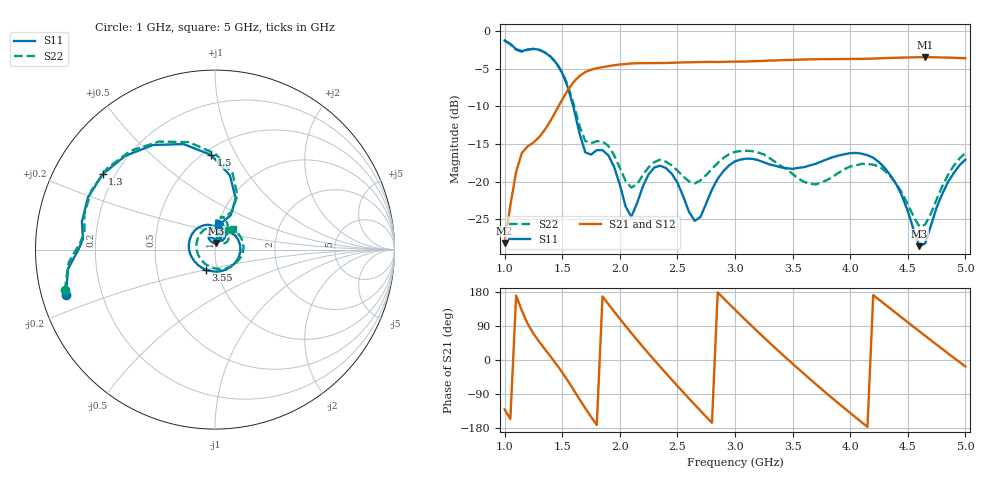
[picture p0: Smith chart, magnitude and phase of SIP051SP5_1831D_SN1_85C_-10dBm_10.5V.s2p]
# GHz  S  dB  R  50
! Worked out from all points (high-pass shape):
!   81 points, 1 GHz to 5 GHz, reference 50 ohm
!   highest |S21| = -3.44 dB at 4.65 GHz (marker M1); lowest = -28.2 dB at 1 GHz (marker M2)
!   |S21| within 3 dB of the highest: 1.618 GHz to end of sweep
!   lowest |S11| = -28.6 dB at 4.6 GHz (marker M3), VSWR 1.08, Z = 50.5 + j3.71 ohm
!   |S11| at or under -10 dB: 1.596 GHz to end of sweep
!   |S22| runs from -26.0 to -1.2 dB; largest |S21 - S12| = 0.002
!   S11 on the Smith chart (normalised r, x): 1 GHz: 0.07, -0.15; 1.3 GHz: 0.15, +0.30; 1.5 GHz: 0.55, +0.80; 3.55 GHz: 0.88, -0.20; 5 GHz: 0.99, +0.28
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1  -1.21 -163.0  -28.17 -130.3  -28.21 -130.4  -1.24 -164.9
1.15  -2.64 175.4  -16.18 129.9  -16.16 130.0  -2.71 172.8
1.3  -2.45 146.1  -14.08 48.2  -14.09 48.2  -2.47 142.9
1.5  -5.55 92.3  -9.08 -32.6  -9.06 -32.7  -5.44 89.8
1.7  -16.09 75.4  -5.42 -127.1  -5.41 -127.2  -14.57 73.1
1.85  -15.81 81.9  -4.76 167.8  -4.75 167.9  -14.67 75.0
2.05  -23.28 68.8  -4.36 89.9  -4.34 89.9  -19.88 63.5
2.2  -20.64 109.1  -4.23 34.8  -4.23 34.9  -19.12 86.2
2.35  -17.88 83.7  -4.22 -17.6  -4.20 -17.6  -17.08 71.2
2.6  -24.00 51.2  -4.12 -101.4  -4.11 -101.4  -19.96 53.7
2.8  -21.06 79.0  -4.07 -165.7  -4.05 -165.8  -18.29 59.2
3  -17.29 36.4  -4.03 132.8  -4.02 132.8  -16.04 32.5
3.25  -17.43 -32.7  -3.93 59.7  -3.92 59.7  -16.38 -14.4
3.4  -18.09 -75.8  -3.83 17.6  -3.83 17.5  -17.93 -48.3
3.55  -18.16 -115.2  -3.77 -23.4  -3.75 -23.5  -19.58 -90.4
3.7  -17.63 -150.1  -3.71 -63.3  -3.71 -63.3  -20.37 -144.7
3.85  -16.74 177.7  -3.69 -102.0  -3.68 -102.1  -19.34 163.4
4.05  -16.18 136.1  -3.67 -152.0  -3.65 -152.1  -17.84 106.6
4.35  -19.18 78.2  -3.54 135.3  -3.54 135.3  -19.31 45.7
4.6  -28.59 80.5  -3.44 75.9  -3.44 75.8  -25.96 47.2
4.65  -28.23 102.9  -3.44 64.0  -3.44 64.0  -25.73 61.8
5  -17.08 83.7  -3.57 -17.0  -3.58 -17.0  -16.19 49.1
